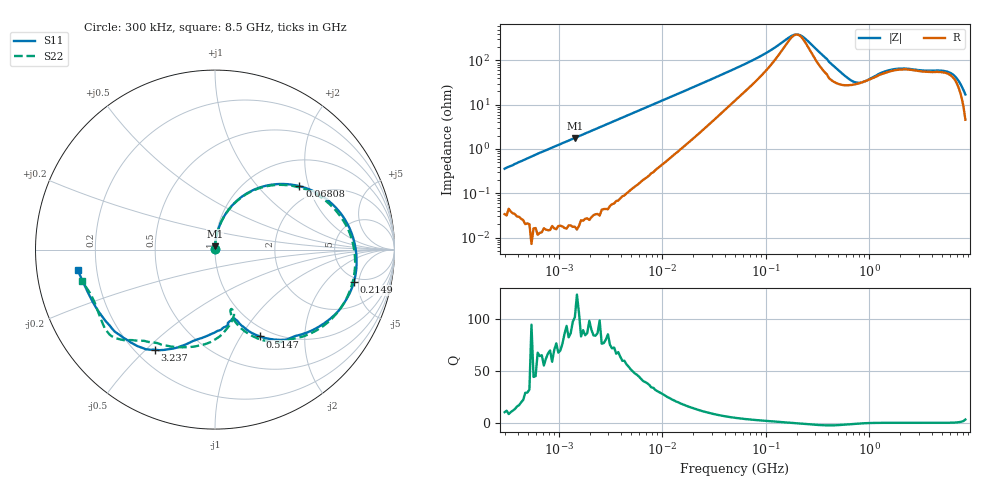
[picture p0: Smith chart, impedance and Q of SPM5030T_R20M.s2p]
! S-Parameter Data Generated by TDK Corporation
! Copyright(C) 2023 TDK Corporation.
! All Rights Reserved.
! TDK P/N: SPM5030T-R20M (Inductor)
! Property: L=200nH at 100kHz
! Size(LxWxT): 5.2x5x3mm
! Model Type: s2p (Touchstone File Format Version 1.0)
! Frequency: DC=Yes Start=0.3MHz Stop=8500MHz 225points Log-sweep
! Model Generated on Sep. 29, 2023
! Port Assignments:
!  1 ---@@@--- 2
! Applicable Conditions:
!  Temperature = 25 degC
!  DC Bias Current = 0 A
!  Small Signal Operation
! Terms and conditions regarding TDK Simulation Models
! (1)This simulation model is being provided solely for informational purposes. Please refer to the specifications of the products in terms of detailed characteristics of such products.
! (2)In no event shall TDK Corporation of any of its subsidiaries be liable for any loss or damage arising, directly or indirectly,
!  From any information contained in this simulation model, including, but not limited to loss or damages arising from any inaccuracies, omissions or errors in connection with such information.
! (3)Any and all copyrights on this simulation model are owned by TDK Corporation.
!  Duplication or redistribution of this simulation model without prior written permission from TDK Corporation is prohibited.
! (4)This simulation model is subject to any modification or change without any prior notice.
! (5)Neither TDK Corporation nor any of its subsidiaries shall make any warranty, express or implied,
!  Including but not limited to the correctness, implied warranties of merchantability and fitness for a particular purpose with respect to this simulation models.
! (6)The use of this simulation model shall be deemed to have consented to the terms and conditions hereof.
# Hz S MA R 50
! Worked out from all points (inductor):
!   224 points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, 300 kHz to 8.5 GHz, reference 50 ohm
!   read as one part in series: L = 194 nH near 314.1 kHz
!   highest Q = 102 at 1.432 MHz (marker M1), where L = 198 nH
!   self-resonance near 199.7 MHz
!   S11 on the Smith chart (normalised r, x): 300 kHz: 1.00, +0.01; 68.08 MHz: 1.61, +1.74; 214.9 MHz: 4.42, -4.31; 514.7 MHz: 0.88, -1.21; 3.237 GHz: 0.28, -0.53; 8.5 GHz: 0.13, -0.07
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300000  0.004127 92.0  1 -0.3  0.9982 -0.1  0.004242 94.3
1432013  0.0174 88.6  0.9998 -1.1  0.9993 -1.0  0.01741 88.7
1721110  0.02082 88.2  0.9997 -1.3  0.9991 -1.2  0.02085 88.3
9430415  0.1118 81.0  0.9897 -7.0  0.9896 -6.8  0.112 81.0
2.476313e7  0.2807 67.4  0.9344 -17.6  0.9343 -17.4  0.2807 67.1
5.167171e7  0.5008 46.7  0.7712 -32.0  0.7712 -31.8  0.4993 46.2
6.808408e7  0.5886 36.9  0.6669 -37.9  0.6671 -37.8  0.5853 36.2
1.356836e8  0.759 9.0  0.333 -43.1  0.3329 -43.0  0.7531 7.9
1.787805e8  0.7906 -3.8  0.2182 -24.5  0.2183 -24.4  0.7842 -5.3
2.148731e8  0.7945 -13.1  0.2093 2.3  0.2093 2.4  0.7874 -14.8
2.831228e8  0.7598 -28.5  0.3299 24.2  0.3298 24.4  0.7563 -30.5
3.906008e8  0.6571 -47.1  0.5218 18.9  0.5217 19.1  0.6543 -49.7
5.146664e8  0.5447 -62.7  0.6559 4.1  0.6559 4.2  0.5269 -66.4
6.47669e8  0.4612 -69.7  0.6989 -9.1  0.6989 -9.0  0.4277 -73.9
8.150429e8  0.4072 -73.5  0.6957 -22.5  0.6958 -22.4  0.3636 -76.0
1.124446e9  0.4097 -79.0  0.6211 -41.3  0.6214 -41.2  0.3543 -73.9
1.551304e9  0.4632 -90.5  0.4983 -57.1  0.4983 -56.9  0.4326 -79.6
2.24089e9  0.5376 -105.3  0.3882 -70.9  0.3883 -70.8  0.5528 -102.1
3.237012e9  0.6508 -121.0  0.3128 -89.4  0.3128 -89.1  0.6233 -124.1
6.161135e9  0.7235 -144.3  0.1791 -119.0  0.1798 -118.6  0.7543 -144.5
7.072242e9  0.7362 -152.8  0.1722 -127.1  0.1721 -126.8  0.7368 -152.3
8.5e9  0.7734 -171.6  0.1408 -143.3  0.1413 -143.4  0.764 -166.7
